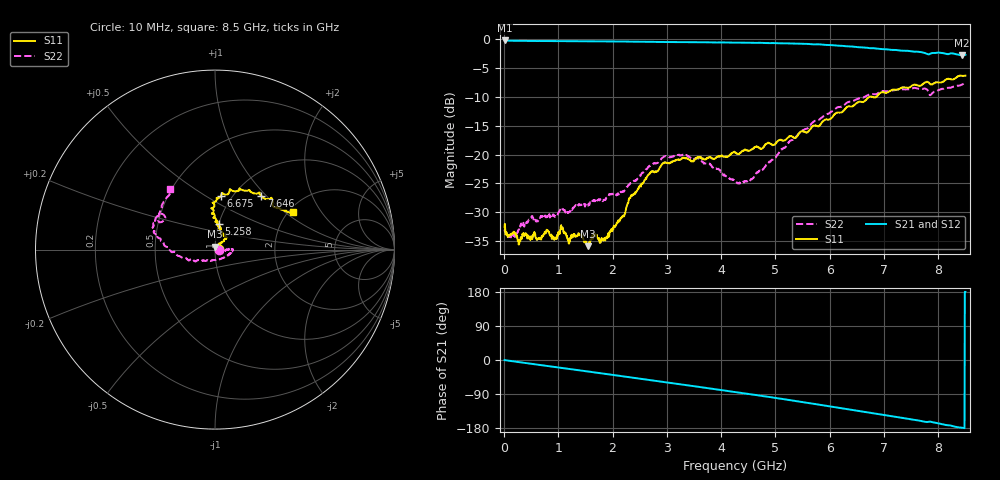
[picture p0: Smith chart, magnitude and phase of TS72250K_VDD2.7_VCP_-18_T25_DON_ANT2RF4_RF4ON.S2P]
!Agilent Technologies,E5071C,MY46417908,A.11.23
!Date: Thu Oct 03 13:34:05 2019
!Data & Calibration Information:
!Freq	S11:SOLT2(ON)	S21:SOLT2(ON)	S12:SOLT2(ON)	S22:SOLT2(ON)
!PortZ  Port1:50+j0  Port2:50+j0
!Above PortZ is port z conversion or system Z0 setting when saving the data.
!When reading, reference impedance value at option line is always used.
# Hz S dB R 50
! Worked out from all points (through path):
!   1601 points, 10 MHz to 8.5 GHz, reference 50 ohm
!   highest |S21| = -0.22 dB at 10 MHz (marker M1); lowest = -2.7 dB at 8.431 GHz (marker M2)
!   group delay of S21, straight-line fit = 58.4 ps
!   lowest |S11| = -35.9 dB at 1.549 GHz (marker M3), VSWR 1.03, Z = 49.9 + j1.6 ohm
!   |S11| at or under -10 dB: start of sweep to 6.739 GHz; 6.783 GHz to 6.861 GHz (78.2 MHz wide, 1.15 % of centre)
!   |S22| runs from -34.3 to -7.5 dB; largest |S21 - S12| = 0.0045
!   S11 on the Smith chart (normalised r, x): 10 MHz: 1.05, +0.01; 5.258 GHz: 1.01, +0.29; 6.675 GHz: 0.89, +0.58; 7.646 GHz: 1.32, +0.93; 8.5 GHz: 2.12, +1.15
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1e7  -32.59 12.1  -0.22 -0.2  -0.24 -0.2  -33.32 -8.8
2.85925e8  -35.12 25.1  -0.29 -5.8  -0.30 -5.8  -32.54 14.1
7.900188e8  -33.16 47.4  -0.33 -15.6  -0.33 -15.6  -30.80 20.0
9.332875e8  -34.45 56.9  -0.34 -18.4  -0.35 -18.4  -30.73 14.5
1.07125e9  -32.81 63.1  -0.35 -21.1  -0.35 -21.1  -29.24 10.8
1.187988e9  -35.20 69.0  -0.35 -23.4  -0.35 -23.4  -30.01 3.0
1.426769e9  -34.02 82.4  -0.37 -28.0  -0.38 -28.0  -28.73 -8.1
1.548812e9  -35.89 91.1  -0.37 -30.4  -0.38 -30.4  -28.71 -19.3
1.899025e9  -34.49 84.0  -0.40 -37.3  -0.40 -37.3  -27.47 -24.9
2.339444e9  -27.08 51.4  -0.43 -46.0  -0.44 -46.1  -24.93 -4.8
2.843538e9  -22.71 47.1  -0.48 -56.0  -0.48 -56.1  -21.31 1.2
3.337019e9  -20.66 47.8  -0.52 -66.0  -0.52 -66.0  -20.09 -2.2
4.255e9  -19.62 70.0  -0.60 -84.5  -0.62 -84.5  -24.66 -65.4
4.557456e9  -19.13 72.6  -0.63 -90.7  -0.63 -90.8  -24.25 -102.8
5.257881e9  -16.82 80.7  -0.75 -105.6  -0.74 -105.6  -17.76 -150.0
5.671769e9  -15.23 89.0  -0.88 -115.0  -0.88 -114.9  -14.56 -166.1
6.67465e9  -10.47 83.7  -1.48 -137.7  -1.50 -137.8  -9.85 168.3
7.088538e9  -9.12 69.0  -1.80 -147.0  -1.81 -147.1  -9.02 163.1
7.645694e9  -8.08 49.1  -2.20 -159.9  -2.17 -159.8  -8.62 155.1
7.94815e9  -7.51 33.3  -2.39 -165.6  -2.38 -165.6  -9.01 153.2
8.431019e9  -6.35 27.3  -2.74 -178.6  -2.76 -178.7  -7.90 128.1
8.5e9  -6.33 25.5  -2.72 179.6  -2.75 179.4  -7.54 126.8
